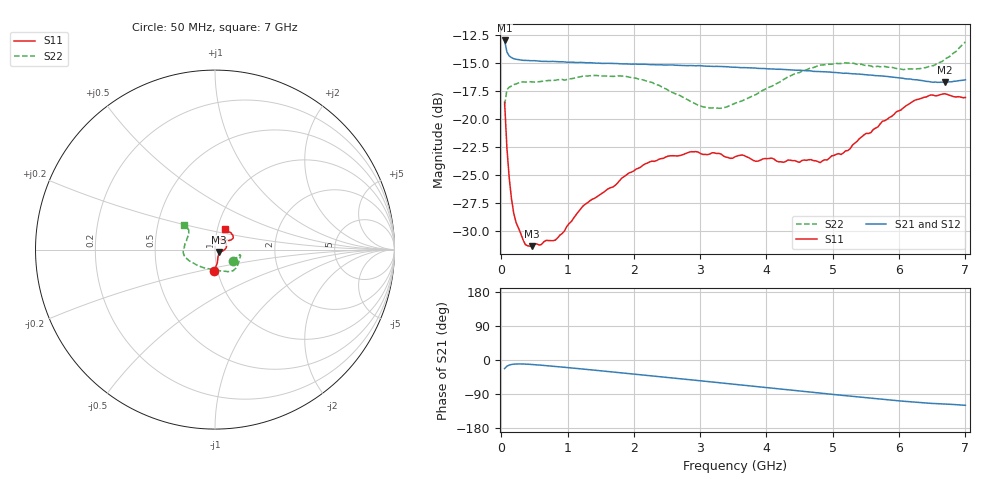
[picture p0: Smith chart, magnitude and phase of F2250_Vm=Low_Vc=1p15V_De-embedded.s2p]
! Integrated Device Technology
! Corporate Headquarters
! 6024 Silver Creek Valley Road
! San Jose, CA 95138  USA
! Phone:  1-408-284-8200
! Toll Free:  1-800-223-1366
! Webpage:  http://www.idt.com/
! Timing and RF Division
! 515 Groton Road, Suite 102
! Westford, MA 01886-6024
! Device:  F2250
! Description: Voltage Variable RF Attenuator
! Frequency:  50.0 -  6000.00 MHz
! Package:  3x3 mm Thin QFN Plastic Package: 16 pin
! Ports:  2 RF, 3 DC
!  Pin  1  = GND
!  Pin  2  = NC
!  Pin  3  = RF1  = Port 1
!  Pin  4  = NC
!  Pin  5  = GND
!  Pin  6  = GND
!  Pin  7  = GND
!  Pin  8  = GND
!  Pin  9  = NC
!  Pin 10  = RF2  = Port 2
!  Pin 11  = NC
!  Pin 12  = GND
!  Pin 13  = GND
!  Pin 14  = VCNTRL
!  Pin 15  = VDD
!  Pin 16  = VMODE
! Vcntrl:  1.150 Volts
! Vmode:  +0.000 Volts
! Vdd:  +3.30  Volts
! Current:  1.193 mA
! Data:  The device was measured on a the F2250 evaluation board which has
!  individual transmission lines to the RF pins.  Data was collected
!  using a calibrated network analyzer.  The evaluation board was
!  de-embedded using a TRL calibration technique.
!  The reference plane is the edge of the package pin.
! Misc:  SN 10
!  Action Tracker AT0258
! Date Measured:  2014-11-26
! Date:  2015-10-15  MJV
! Note:
!  Integrated Device Technology supplies this data as a sample of measured
!  data at the package pin for this product.  Your particular data for this
!  product may vary.
!  Data was taken at 25 degrees C.
!  Integrated Device Technology reserves the right to change this data at anytime.
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# GHz S dB R 50
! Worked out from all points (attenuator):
!   201 points, 50 MHz to 7 GHz, reference 50 ohm
!   highest |S21| = -13.00 dB at 50 MHz (marker M1); lowest = -16.7 dB at 6.687 GHz (marker M2)
!   lowest |S11| = -31.3 dB at 467 MHz (marker M3), VSWR 1.06, Z = 52.4 - j1.45 ohm
!   |S11| at or under -10 dB: start of sweep to end of sweep
!   |S22| runs from -19.0 to -13.1 dB; largest |S21 - S12| = 0.00059
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0.05  -18.50 -91.9  -13.00 -22.6  -13.00 -22.6  -18.76 -31.9
0.08475  -22.60 -79.8  -14.02 -16.4  -14.02 -16.4  -17.39 -16.7
0.1195  -25.25 -73.4  -14.38 -13.3  -14.37 -13.3  -17.17 -12.7
0.189  -28.45 -60.7  -14.62 -10.9  -14.63 -10.9  -16.93 -11.4
0.36275  -31.20 -37.0  -14.77 -10.8  -14.76 -10.8  -16.71 -13.5
0.467  -31.35 -30.8  -14.80 -11.9  -14.80 -11.9  -16.70 -15.8
0.8145  -30.81 -17.9  -14.88 -17.0  -14.88 -17.0  -16.55 -26.2
1.2315  -27.78 -12.8  -14.96 -23.9  -14.96 -23.9  -16.19 -36.8
1.89175  -24.98 2.5  -15.09 -35.2  -15.10 -35.2  -16.22 -49.6
2.37825  -23.59 14.6  -15.17 -43.7  -15.16 -43.7  -17.00 -60.4
2.86475  -22.92 30.1  -15.24 -52.4  -15.23 -52.4  -18.46 -78.9
3.0385  -23.16 36.5  -15.27 -55.5  -15.28 -55.5  -18.91 -88.2
3.3165  -23.14 46.6  -15.31 -60.5  -15.32 -60.5  -19.04 -105.9
3.525  -23.37 52.3  -15.39 -64.2  -15.38 -64.3  -18.60 -119.0
3.83775  -23.77 62.5  -15.46 -69.8  -15.46 -69.8  -17.83 -135.5
4.7065  -23.71 63.3  -15.75 -85.4  -15.74 -85.5  -15.42 -164.8
4.81075  -23.90 59.4  -15.77 -87.3  -15.78 -87.3  -15.19 -166.6
5.1235  -23.17 49.7  -15.90 -92.9  -15.89 -92.9  -15.05 -173.7
5.85325  -19.87 31.4  -16.22 -105.4  -16.23 -105.5  -15.40 169.8
6.2355  -18.33 33.0  -16.50 -111.4  -16.50 -111.4  -15.55 157.1
6.68725  -17.75 45.7  -16.74 -116.2  -16.73 -116.2  -14.66 143.0
7  -18.08 64.3  -16.50 -119.6  -16.49 -119.7  -13.12 141.6
